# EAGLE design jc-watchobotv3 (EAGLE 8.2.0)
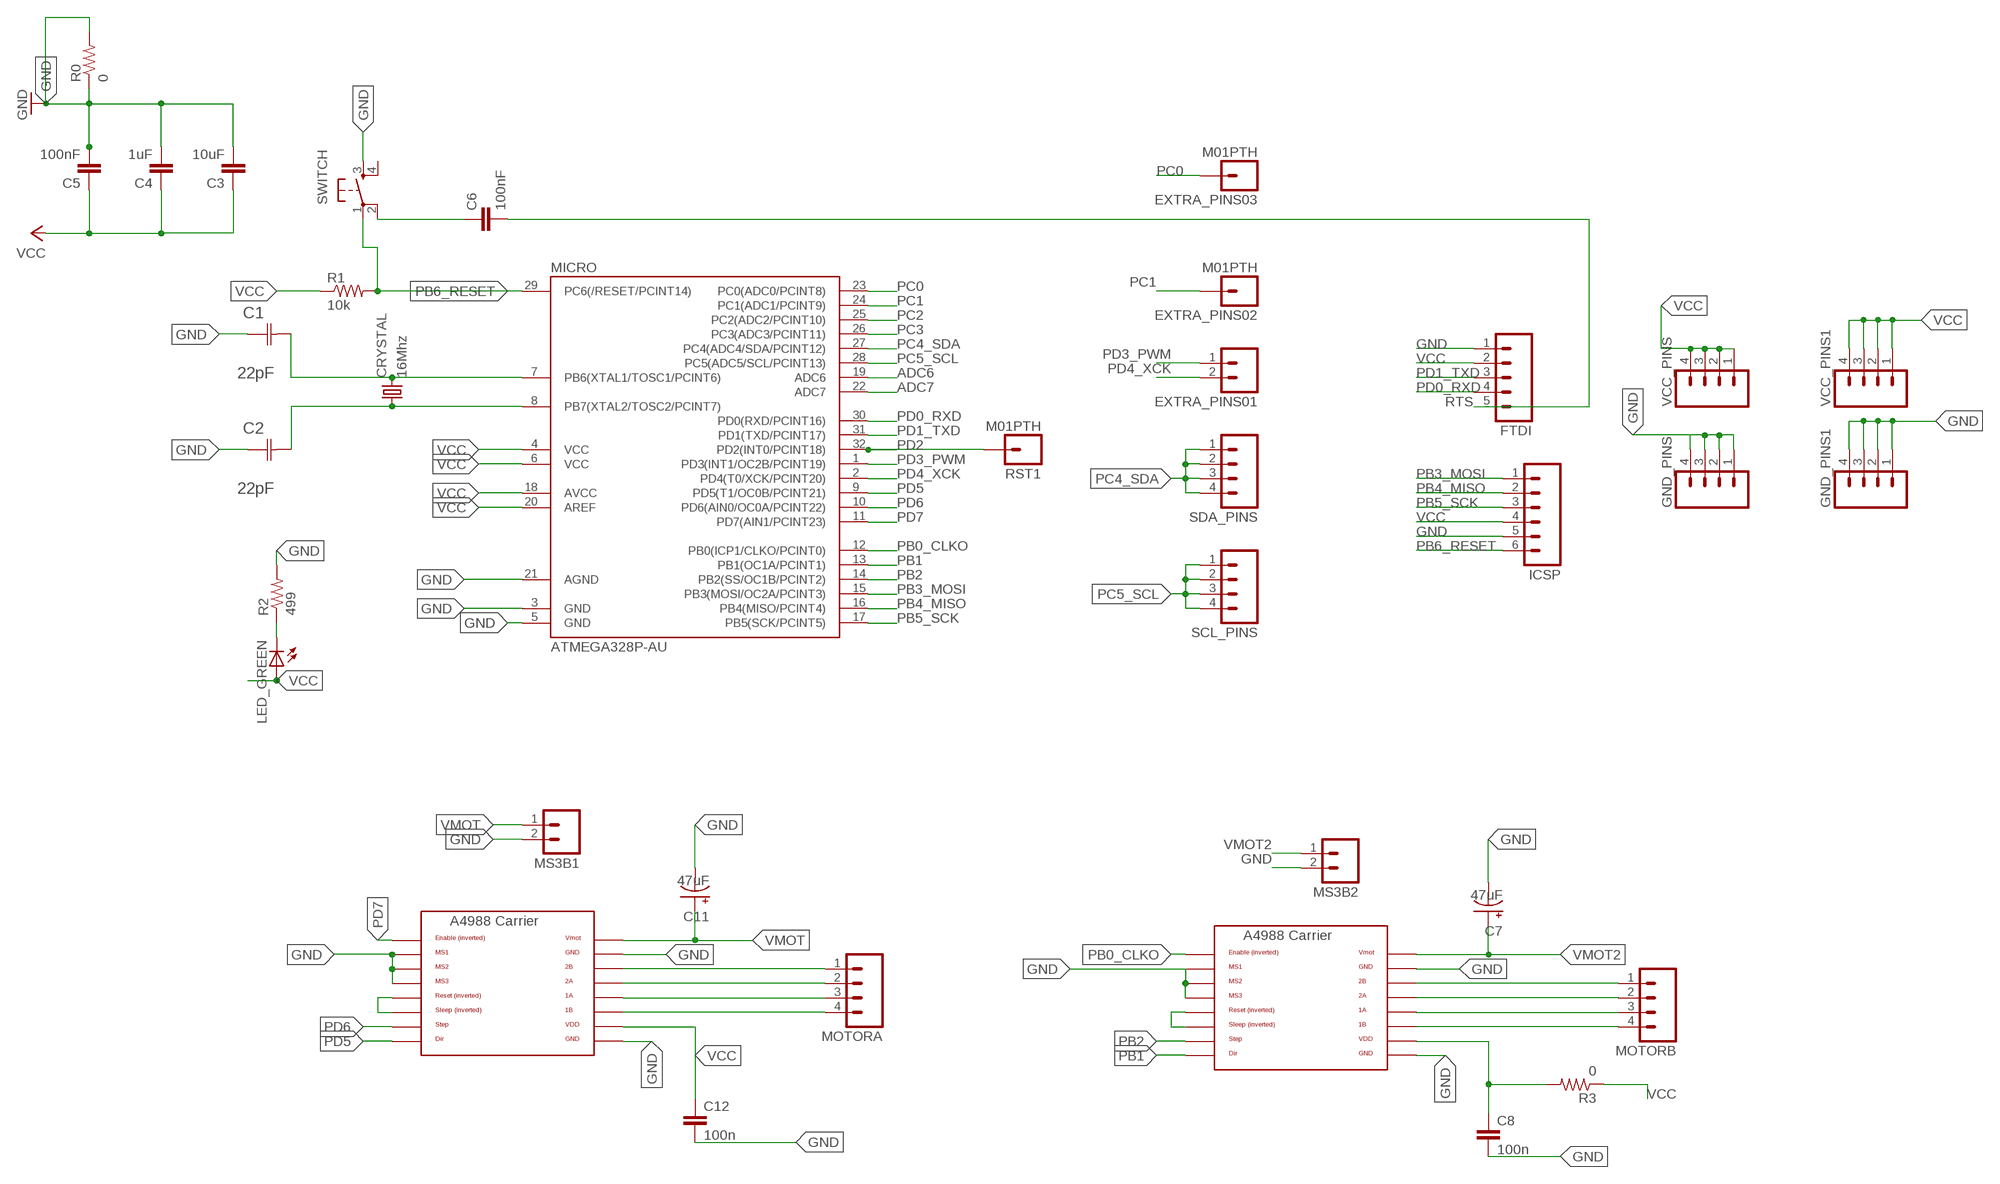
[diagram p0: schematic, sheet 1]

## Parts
C1  22pF  0612ZC225MAT2A  [CAPC3216X178N]
C2  22pF  0612ZC225MAT2A  [CAPC3216X178N]
C3  10uF  CAP1206  [1206]
C4  1uF  CAP1206  [1206]
C5  100nF  CAP1206  [1206]
C6  100nF  CAP1206  [1206]
C7  47uF  MCGPR50V107M8X11  [MCGPR50V107M8X11]
C8  100n  CAP1206  [1206]
C11  47uF  MCGPR50V107M8X11  [MCGPR50V107M8X11]
C12  100n  CAP1206  [1206]
CRYSTAL  16Mhz  CSM-7X-DU  [CSM-7X-DU]
EXTRA_PINS01  M02  [02P]
EXTRA_PINS02  M01PTH  [1X01]
EXTRA_PINS03  M01PTH  [1X01]
FTDI  M05  [05P]
GND_PINS  M04  [04P]
GND_PINS1  M04  [04P]
ICSP  M06  [06P]
LED_GREEN  LED1206  [1206]
MICRO  ATMEGA328P-AU  ATMEGA48/88/168-AU  [TQFP32-08]
MOTORA  M04  [04P]
MOTORA_CARRIER  A4988BREAKOUT  [A4988BREAKOUT]
MOTORB  M04  [04P]
MOTORB_CARRIER  A4988BREAKOUT  [A4988BREAKOUT]
MS3B1  M02  [02P]
MS3B2  M02  [02P]
R0  0  RESISTOR1206  [1206]
R1  10k  RESISTOR1206  [1206]
R2  499  RESISTOR1206  [1206]
R3  0  RESISTOR1206  [1206]
RST1  M01PTH  [1X01]
SCL_PINS  M04  [04P]
SDA_PINS  M04  [04P]
SWITCH  6MM_SWITCH6MM_SWITCH  [6MM_SWITCH]
VCC_PINS  M04  [04P]
VCC_PINS1  M04  [04P]

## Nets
ADC6: MICRO.19(ADC6)
ADC7: MICRO.22(ADC7)
GND: C1.1(C1) C2.1(C1) C3.2 C4.2 C5.2 C7.- C8.2 C11.- C12.2 FTDI.1 GND_PINS1.1 GND_PINS1.2 GND_PINS1.3 GND_PINS1.4 GND_PINS.1 GND_PINS.2 GND_PINS.3 GND_PINS.4 ICSP.5 MICRO.3(GND) MICRO.5(GND) MICRO.21(AGND) MOTORA_CARRIER.GND MOTORA_CARRIER.GND@0(GND) MOTORA_CARRIER.MS1 MOTORA_CARRIER.MS2 MOTORA_CARRIER.MS3 MOTORB_CARRIER.GND MOTORB_CARRIER.GND@0(GND) MOTORB_CARRIER.MS1 MOTORB_CARRIER.MS2 MOTORB_CARRIER.MS3 MS3B1.2 MS3B2.2 R0.1 R0.2 R2.2 SWITCH.3(S)
N$6: MOTORA_CARRIER.RST MOTORA_CARRIER.SLP(SLEEP)
N$9: MOTORB_CARRIER.RST MOTORB_CARRIER.SLP(SLEEP)
N$11: MOTORA.1 MOTORA_CARRIER.2B
N$12: MOTORA.2 MOTORA_CARRIER.2A
N$13: MOTORA.3 MOTORA_CARRIER.1A
N$14: MOTORA.4 MOTORA_CARRIER.1B
N$16: MOTORB.1 MOTORB_CARRIER.2B
N$17: MOTORB.2 MOTORB_CARRIER.2A
N$18: MOTORB.3 MOTORB_CARRIER.1A
N$19: MOTORB.4 MOTORB_CARRIER.1B
N$22: C6.1 SWITCH.2(P1)
N$26: LED_GREEN.2(C) R2.1
PB0_CLKO: MICRO.12(PB0(ICP1/CLKO/PCINT0)) MOTORB_CARRIER.EN
PB1: MICRO.13(PB1(OC1A/PCINT1)) MOTORB_CARRIER.DIR
PB2: MICRO.14(PB2(SS/OC1B/PCINT2)) MOTORB_CARRIER.STEP
PB3_MOSI: ICSP.1 MICRO.15(PB3(MOSI/OC2A/PCINT3))
PB4_MISO: ICSP.2 MICRO.16(PB4(MISO/PCINT4))
PB5_SCK: ICSP.3 MICRO.17(PB5(SCK/PCINT5))
PB6_RESET: ICSP.6 MICRO.29(PC6(/RESET/PCINT14)) R1.2 SWITCH.1(P)
PB6_XTAL1: C1.2(C2) CRYSTAL.2 MICRO.7(PB6(XTAL1/TOSC1/PCINT6))
PB7_XTAL2: C2.2(C2) CRYSTAL.1 MICRO.8(PB7(XTAL2/TOSC2/PCINT7))
PC0: EXTRA_PINS03.1 MICRO.23(PC0(ADC0/PCINT8))
PC1: EXTRA_PINS02.1 MICRO.24(PC1(ADC1/PCINT9))
PC2: MICRO.25(PC2(ADC2/PCINT10))
PC3: MICRO.26(PC3(ADC3/PCINT11))
PC4_SDA: MICRO.27(PC4(ADC4/SDA/PCINT12)) SDA_PINS.1 SDA_PINS.2 SDA_PINS.3 SDA_PINS.4
PC5_SCL: MICRO.28(PC5(ADC5/SCL/PCINT13)) SCL_PINS.1 SCL_PINS.2 SCL_PINS.3 SCL_PINS.4
PD0_RXD: FTDI.4 MICRO.30(PD0(RXD/PCINT16))
PD1_TXD: FTDI.3 MICRO.31(PD1(TXD/PCINT17))
PD2: MICRO.32(PD2(INT0/PCINT18)) RST1.1
PD3_PWM: EXTRA_PINS01.1 MICRO.1(PD3(INT1/OC2B/PCINT19))
PD4_XCK: EXTRA_PINS01.2 MICRO.2(PD4(T0/XCK/PCINT20))
PD5: MICRO.9(PD5(T1/OC0B/PCINT21)) MOTORA_CARRIER.DIR
PD6: MICRO.10(PD6(AIN0/OC0A/PCINT22)) MOTORA_CARRIER.STEP
PD7: MICRO.11(PD7(AIN1/PCINT23)) MOTORA_CARRIER.EN
RTS: C6.2 FTDI.5
VCC: C3.1 C4.1 C5.1 C8.1 C12.1 FTDI.2 ICSP.4 LED_GREEN.1(A) MICRO.4(VCC) MICRO.6(VCC) MICRO.18(AVCC) MICRO.20(AREF) MOTORA_CARRIER.VDD MOTORB_CARRIER.VDD R1.1 R3.1 R3.2 VCC_PINS1.1 VCC_PINS1.2 VCC_PINS1.3 VCC_PINS1.4 VCC_PINS.1 VCC_PINS.2 VCC_PINS.3 VCC_PINS.4
VMOT: C11.+ MOTORA_CARRIER.VMOT MS3B1.1
VMOT2: C7.+ MOTORB_CARRIER.VMOT MS3B2.1
Unconnected: SWITCH.4(S1)

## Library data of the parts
C1 C2 = AVX_By_element14_Batch_1:0612ZC225MAT2A: Capacitor 1206; MPN: 0612ZC225MAT2A; OC_FARNELL: -; OC_NEWARK: 12N3209; SUPPLIER: AVX; TOLERANCE: ±20%; VALUE: 2.2µF; VOLTAGERATING: 10V
C3-C6 C8 C12 = 01_SparkFun:CAP: Capacitor
C7 C11 = Ryan:MCGPR50V107M8X11
CRYSTAL = 01_FAB_Hello:CSM-7X-DU: SMD CRYSTAL; OC_FARNELL: unknown; OC_NEWARK: unknown
EXTRA_PINS01 MS3B1 MS3B2 = con-amp-quick:M02: AMP QUICK CONNECTOR; OC_FARNELL: unknown; OC_NEWARK: unknown
EXTRA_PINS02 EXTRA_PINS03 RST1 = 01_SparkFun:M01: Header 1
FTDI = con-amp-quick:M05: AMP QUICK CONNECTOR; OC_FARNELL: unknown; OC_NEWARK: unknown
GND_PINS GND_PINS1 MOTORA MOTORB SCL_PINS SDA_PINS VCC_PINS VCC_PINS1 = con-amp-quick:M04: AMP QUICK CONNECTOR; OC_FARNELL: unknown; OC_NEWARK: unknown
ICSP = con-amp-quick:M06: AMP QUICK CONNECTOR; OC_FARNELL: unknown; OC_NEWARK: unknown
LED_GREEN = 01_FAB_Hello:LED
MICRO = atmega8:ATMEGA48/88/168
MOTORA_CARRIER MOTORB_CARRIER = RepRapjr:A4988BREAKOUT
R0 R1-R3 = 01_SparkFun:RESISTOR: Resistor
SWITCH = 01_FAB_Hello:6MM_SWITCH: OMRON SWITCH

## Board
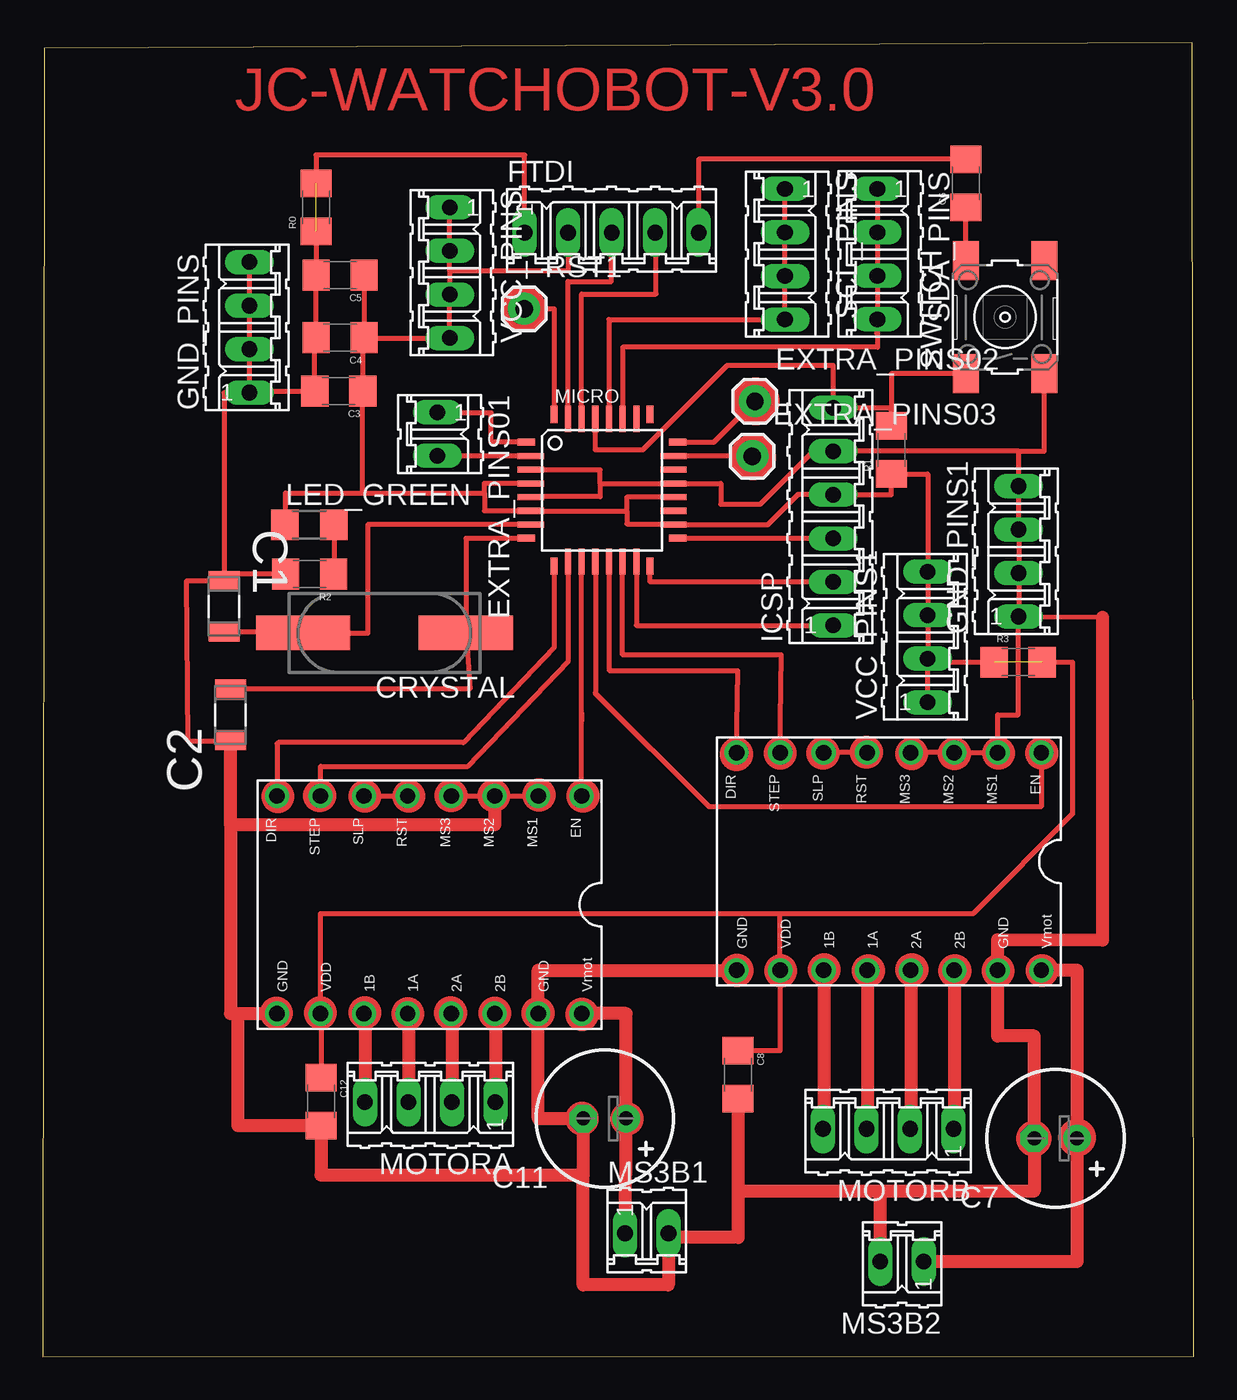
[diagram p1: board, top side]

Size 67.16 x 76.66 mm. Coordinates in mm from the lower left corner, seen from the top.
Outline: 0,0 67.16,0.02 67.08,76.66 0.09,76.36 0,0
Copper layers (1*16): Top 0.035mm / dielectric 1.5mm / Bottom 0.035mm
Design rules "default *": minimum track width 10mil, minimum drill 24mil, track to track 8mil, track to pad 8mil, pad to pad 8mil, via to via 8mil, smd to smd 8mil, copper to edge 40mil, drill to drill 8mil, minimum pad ring 10mil, minimum via ring 8mil, stop-mask expansion 4mil, vias tented up to drill 0mil, thermal gap 10mil

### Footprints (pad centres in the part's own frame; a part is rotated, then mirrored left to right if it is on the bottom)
CAPC3216X178N = smd 1.118 x 1.803: 1 -1.499,0; 2 1.499,0
1206 = smd 1.6 x 1.8: 1 -1.4,0; 2 1.4,0
MCGPR50V107M8X11 = drill 0.813 pad 1.6: + -1.25,0 | drill 0.813 pad 1.6 octagon: - 1.25,0
CSM-7X-DU = smd 5.5 x 2: 1 -4.75,0; 2 4.75,0
02P = drill 0.914 long: 1 -1.27,0; 2 1.27,0
1X01 = drill 1.016 pad 1.88: 1 0,0
05P = drill 0.914 long: 1 -5.08,0; 2 -2.54,0; 3 0,0; 4 2.54,0; 5 5.08,0
04P = drill 0.914 long: 1 -3.81,0; 2 -1.27,0; 3 1.27,0; 4 3.81,0
06P = drill 0.914 long: 1 -6.35,0; 2 -3.81,0; 3 -1.27,0; 4 1.27,0; 5 3.81,0; 6 6.35,0
1206' = smd 1.6 x 1.803: 1 -1.422,0; 2 1.422,0
TQFP32-08 = smd 1.016 x 0.406: 1 -4.42,2.8; 8 -4.42,-2.8; 17 4.42,-2.8; 24 4.42,2.8 | smd 1.524 x 0.356: 2 -4.166,2; 3 -4.166,1.2; 4 -4.166,0.4; 5 -4.166,-0.4; 6 -4.166,-1.2; 7 -4.166,-2; 18 4.166,-2; 19 4.166,-1.2; 20 4.166,-0.4; 21 4.166,0.4; 22 4.166,1.2; 23 4.166,2 | smd 0.406 x 1.016: 9 -2.8,-4.42; 16 2.8,-4.42; 25 2.8,4.42; 32 -2.8,4.42 | smd 0.356 x 1.524: 10 -2,-4.166; 11 -1.2,-4.166; 12 -0.4,-4.166; 13 0.4,-4.166; 14 1.2,-4.166; 15 2,-4.166; 26 2,4.166; 27 1.2,4.166; 28 0.4,4.166; 29 -0.4,4.166; 30 -1.2,4.166; 31 -2,4.166
A4988BREAKOUT = drill 0.9: 1A 8.89,1.27; 1B 11.43,1.27; 2A 6.35,1.27; 2B 3.81,1.27; DIR 16.51,-11.43; EN -1.27,-11.43; GND 16.51,1.27; GND@0 1.27,1.27; MS1 1.27,-11.43; MS2 3.81,-11.43; MS3 6.35,-11.43; RST 8.89,-11.43; SLP 11.43,-11.43; STEP 13.97,-11.43; VDD 13.97,1.27; VMOT -1.27,1.27
6MM_SWITCH = smd 2.286 x 1.524: 1 -3.302,2.286; 2 3.302,2.286; 3 -3.302,-2.286; 4 3.302,-2.286

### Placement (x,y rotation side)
C1  10.57,43.78 270 top
C2  10.96,37.45 90 top
C3  17.26,56.35 180 top
C4  17.35,59.47 180 top
C5  17.35,63.11 180 top
C6  53.86,68.47 90 top
C7  59.1,12.74 180 top
C8  40.57,16.45 270 top
C11  32.79,13.9 180 top
C12  16.23,14.89 270 top
CRYSTAL  19.94,42.23 180 top
EXTRA_PINS01  23.02,53.84 270 top
EXTRA_PINS02  41.55,55.76 0 top
EXTRA_PINS03  41.4,52.54 0 top
FTDI  33.19,65.59 0 top
GND_PINS  12.05,60.06 90 top
GND_PINS1  56.94,46.99 90 top
ICSP  46.11,49.02 90 top
LED_GREEN  [1206']  15.56,48.54 0 top
MICRO  32.64,50.55 0 top
MOTORA  22.6,14.85 180 top
MOTORA_CARRIER  30.17,21.29 180 top
MOTORB  49.33,13.29 180 top
MOTORB_CARRIER  57,23.81 180 top
MS3B1  35.24,7.19 0 top
MS3B2  50.14,5.54 180 top
R0  15.94,67.06 90 top
R1  49.51,52.91 90 top
R2  15.57,45.66 180 top
R3  56.91,40.52 0 top
RST1  28.09,61.15 0 top
SCL_PINS  43.31,64.33 270 top
SDA_PINS  48.7,64.34 270 top
SWITCH  56.15,60.66 90 top
VCC_PINS  23.75,63.25 270 top
VCC_PINS1  51.63,41.99 90 top

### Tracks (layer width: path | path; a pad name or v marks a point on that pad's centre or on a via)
GND  (1 unrouted)
  Top 0.305: MICRO.3 32.52,51.75 32.52,50.95 | 32.52,50.95 32.52,50.18 28.47,50.18 MICRO.5 | 32.52,50.95 MICRO.21 39.56,50.95 39.56,49.74 41.87,49.74 44.91,52.78 46.07,52.78 ICSP.5 56.94,52.83 | SWITCH.3 58.43,52.83 56.94,52.83 | GND_PINS1.1 GND_PINS1.2 GND_PINS1.3 GND_PINS1.4 56.94,52.83 | MOTORB_CARRIER.MS3 MOTORB_CARRIER.MS2 MOTORB_CARRIER.MS1 55.73,37.45 56.92,37.45 56.92,43.18 GND_PINS1.1 | 57.86,12.74 C7.- | 57.85,18.71 57.9,18.71 | FTDI.1 28.11,70.12 15.94,70.12 R0.2 | R0.1 15.95,65.66 C5.2 C4.2 15.86,59.47 C3.2 12.05,56.35 GND_PINS.1 | GND_PINS.4 GND_PINS.3 GND_PINS.2 GND_PINS.1 | GND_PINS.1 11.46,56.25 | R2.2 10.57,45.66 C1.1 | GND_PINS.1 10.57,56.25 C1.1 | C1.1 8.4,45.28 8.49,35.91 10.71,35.91 C2.1 | MOTORA_CARRIER.MS3 MOTORA_CARRIER.MS2 MOTORA_CARRIER.MS1 | GND_PINS1.1 61.85,43.15 | 10.96,20.02 11.39,20.02 | 36.57,6.96 MS3B1.2 | 31.54,10.59 31.53,10.59
  Top 0.762: MS3B2.2 48.87,9.65 | 48.87,9.65 40.57,9.65 | 48.87,9.65 57.85,9.65 C7.- 57.85,18.71 55.73,18.71 MOTORB_CARRIER.GND@0 55.73,24.34 61.85,24.31 61.85,43.15 | C8.2 40.57,9.65 | 10.96,31.03 C2.1 | 10.96,31.03 10.96,20.02 | MOTORA_CARRIER.MS2 26.36,31.03 10.96,31.03 | MOTORB_CARRIER.GND 28.9,22.54 MOTORA_CARRIER.GND@0 28.9,13.9 C11.- 31.54,10.59 | MOTORA_CARRIER.GND 11.39,20.02 11.39,13.49 C12.2 16.23,10.59 31.53,10.59 31.53,4.19 36.51,4.19 MS3B1.2 | 36.57,6.96 40.57,6.96 40.57,9.65
N$6
  Top 0.305: MOTORA_CARRIER.SLP MOTORA_CARRIER.RST
N$9
  Top 0.305: MOTORB_CARRIER.RST MOTORB_CARRIER.SLP
N$11
  Top 0.305: MOTORA_CARRIER.2B 26.41,20.02
  Top 0.762: 26.41,20.02 MOTORA.1
N$12
  Top 0.305: MOTORA_CARRIER.2A 23.87,20.02
  Top 0.762: 23.87,20.02 MOTORA.2
N$13
  Top 0.305: MOTORA_CARRIER.1A 21.33,20.02
  Top 0.762: 21.33,20.02 MOTORA.3
N$14
  Top 0.305: MOTORA_CARRIER.1B 18.79,20.02
  Top 0.762: 18.79,20.02 MOTORA.4
N$16
  Top 0.305: 53.19,13.29 MOTORB.1
  Top 0.762: MOTORB_CARRIER.2B 53.19,13.29
N$17
  Top 0.305: 50.65,13.29 MOTORB.2
  Top 0.762: MOTORB_CARRIER.2A 50.65,13.29
N$18
  Top 0.305: 48.11,13.29 MOTORB.3
  Top 0.762: MOTORB_CARRIER.1A 48.11,13.29
N$19
  Top 0.305: 45.57,13.29 MOTORB.4
  Top 0.762: MOTORB_CARRIER.1B 45.57,13.29
N$22
  Top 0.305: SWITCH.2 C6.1
N$26
  Top 0.305: LED_GREEN.2 17,47.17 R2.1
PB0_CLKO
  Top 0.305: MICRO.12 32.24,38.74 32.23,38.74 38.89,32.08 58.27,32.08 MOTORB_CARRIER.EN
PB1
  Top 0.305: MOTORB_CARRIER.DIR 40.56,40.01 33.07,40.01 33.07,46.39 MICRO.13
PB2
  Top 0.305: MICRO.14 33.84,40.95 43.1,40.95 MOTORB_CARRIER.STEP
PB3_MOSI
  Top 0.305: MICRO.15 34.64,42.67 ICSP.1
PB4_MISO
  Top 0.305: ICSP.2 35.44,45.21 MICRO.16
PB5_SCK
  Top 0.305: MICRO.17 ICSP.3
PB6_RESET
  Top 0.305: MICRO.29 32.24,52.93 35.02,52.93 39.94,57.85 46.11,57.85 ICSP.6 49.51,55.37 R1.2 49.51,57.35 SWITCH.1
PB6_XTAL1
  Top 0.305: 14.74,42.28 C1.2 | 14.74,42.28 15.19,42.28 CRYSTAL.2 | MICRO.7 18.96,48.55 18.96,42.2 14.74,42.2 14.74,42.28
PB7_XTAL2
  Top 0.305: MICRO.8 24.69,47.75 CRYSTAL.1 24.92,38.96 C2.2
PC0
  Top 0.305: EXTRA_PINS03.1 36.81,52.54 MICRO.23
PC1
  Top 0.305: MICRO.24 39.15,53.35 EXTRA_PINS02.1
PC4_SDA
  Top 0.305: SDA_PINS.4 48.67,59.71 | SDA_PINS.4 48.7,58.9 33.84,58.9 MICRO.27 | SDA_PINS.1 SDA_PINS.2 SDA_PINS.3 SDA_PINS.4
PC5_SCL
  Top 0.305: MICRO.28 33.04,60.52 SCL_PINS.4 SCL_PINS.3 SCL_PINS.2 SCL_PINS.1
PD0_RXD
  Top 0.305: MICRO.30 31.44,62.01 35.78,62.01 35.78,65.59 FTDI.4
PD1_TXD
  Top 0.305: MICRO.31 30.64,62.73 33.18,62.73 FTDI.3
PD2
  Top 0.305: RST1.1 29.84,61.15 MICRO.32
PD3_PWM
  Top 0.305: MICRO.1 26.16,53.35 26.16,55.06 23.02,55.06 EXTRA_PINS01.1
PD4_XCK
  Top 0.305: MICRO.2 EXTRA_PINS01.2
PD5
  Top 0.305: MOTORA_CARRIER.DIR 13.66,35.75 13.74,35.83 24.55,35.83 29.84,41.38 MICRO.9
PD6
  Top 0.305: MICRO.10 30.64,40.56 24.79,34.45 16.23,34.45 16.2,34.42 | 16.2,34.42 16.2,34.41 | MOTORA_CARRIER.STEP 16.2,34.42
PD7
  Top 0.305: 31.44,37.55 MICRO.11 | 31.44,37.55 31.44,37.1 31.45,37.1 | MOTORA_CARRIER.EN 31.44,37.55
RTS
  Top 0.305: C6.2 38.27,69.87 FTDI.5
VCC  (1 unrouted)
  Top 0.305: MICRO.20 34.09,50.15 34.09,49.35 | 34.09,49.35 34.09,48.59 36.8,48.59 MICRO.18 42.31,48.55 44.08,50.32 46.08,50.32 ICSP.4 49.51,50.29 R1.1 51.63,51.51 VCC_PINS1.4 VCC_PINS1.3 VCC_PINS1.2 | 34.09,49.35 MICRO.6 28.47,49.37 25.77,49.37 25.77,50.4 | MICRO.4 25.77,50.95 25.77,50.4 | VCC_PINS1.1 VCC_PINS1.2 | C5.1 C4.1 | C4.1 18.66,59.47 C3.1 18.66,50.4 | 18.66,50.4 25.77,50.4 | LED_GREEN.1 14.15,50.4 18.66,50.4 | C12.1 16.23,20.02 MOTORA_CARRIER.VDD 16.2,25.85 43.03,25.85 | VCC_PINS1.2 51.63,40.52 R3.1 | R3.2 60.08,40.52 60.08,31.66 60.09,31.65 54.29,25.85 43.03,25.85 | 43.03,25.85 MOTORB_CARRIER.VDD 43.03,17.85 C8.1 | C4.1 18.75,59.44 VCC_PINS.4 VCC_PINS.3 23.75,63.35 | 23.75,63.35 VCC_PINS.2 VCC_PINS.1 | FTDI.2 30.65,63.35 23.75,63.35
VMOT
  Top 0.762: MS3B1.1 33.99,7.19 C11.+ 34.04,20.02 MOTORA_CARRIER.VMOT
VMOT2
  Top 0.762: 58.21,22.54 MOTORB_CARRIER.VMOT 60.35,22.54 C7.+ 60.35,5.54 MS3B2.1
(copper drawn outside any net)
  shapes: Top circle x39

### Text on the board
Top: JC-WATCHOBOT-V3.0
